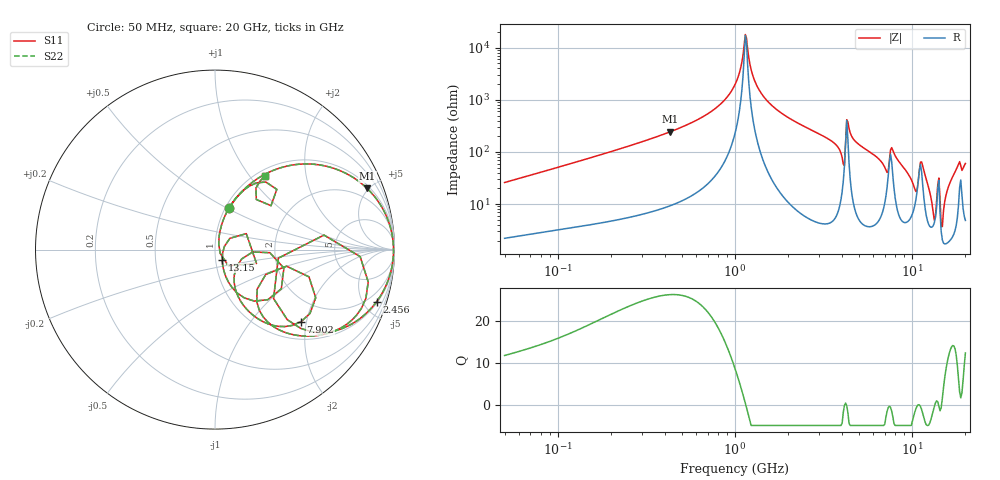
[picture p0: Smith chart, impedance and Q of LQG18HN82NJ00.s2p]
!Murata Part Number: LQG18HN82NJ00
!These Parameters are Measured in Series Mode Connection
!  o--[Z]--o
!Port1  Port2
!  o-------o
!Freq. Start=50[MHz] Stop=20[GHz], 401[Steps]
# Hz S RI R 50
!Freq.(Hz) S11(Real) S11(Imag) S21(Real) S21(Imag) S12(Real) S12(Imag) S22(Real) S22(Imag)
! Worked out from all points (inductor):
!   401 points, 50 MHz to 20 GHz, reference 50 ohm
!   read as one part in series: L = 81.2 nH near 51.52 MHz
!   highest Q = 26.2 at 432.2 MHz (marker M1), where L = 90.1 nH
!   self-resonance near 1.144 GHz
!   S11 on the Smith chart (normalised r, x): 50 MHz: 1.04, +0.52; 2.456 GHz: 1.12, -6.19; 7.902 GHz: 1.41, -1.86; 13.15 GHz: 1.08, -0.12; 20 GHz: 1.10, +1.20
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5e7  0.0802 0.2322  0.9198 -0.2322  0.9198 -0.2322  0.0802 0.2322
1.364002e8  0.3309 0.4439  0.6691 -0.4439  0.6691 -0.4439  0.3309 0.4439
3.721004e8  0.7954 0.3845  0.2046 -0.3845  0.2046 -0.3845  0.7954 0.3845
4.322267e8  0.8479 0.3406  0.1521 -0.3406  0.1521 -0.3406  0.8479 0.3406
1e9  0.9916 0.0499  0.00837 -0.0499  0.00837 -0.0499  0.9916 0.0499
1.161586e9  0.9947 -0.00387  0.00529 0.00387  0.00529 0.00387  0.9947 -0.00387
1.432596e9  0.9886 -0.0804  0.0114 0.0804  0.0114 0.0804  0.9886 -0.0804
2.456456e9  0.9009 -0.2894  0.0991 0.2894  0.0991 0.2894  0.9009 -0.2894
2.728004e9  0.8653 -0.3322  0.1347 0.3322  0.1347 0.3322  0.8653 -0.3322
4.026975e9  0.403 -0.391  0.597 0.391  0.597 0.391  0.403 -0.391
4.275624e9  0.8087 -0.0391  0.1913 0.0391  0.1913 0.0391  0.8087 -0.0391
4.677679e9  0.741 -0.4108  0.259 0.4108  0.259 0.4108  0.741 -0.4108
5.944466e9  0.4661 -0.4792  0.5339 0.4792  0.5339 0.4792  0.4661 -0.4792
7.442007e9  0.3988 -0.0924  0.6012 0.0924  0.6012 0.0924  0.3988 -0.0924
7.901521e9  0.4791 -0.4018  0.5209 0.4018  0.5209 0.4018  0.4791 -0.4018
1.050288e10  0.1188 -0.0988  0.8812 0.0988  0.8812 0.0988  0.1188 -0.0988
1.149051e10  0.2939 -0.2793  0.7061 0.2793  0.7061 0.2793  0.2939 -0.2793
1.314879e10  0.0401 -0.0563  0.9599 0.0563  0.9599 0.0563  0.0401 -0.0563
1.396067e10  0.1744 0.0889  0.8256 -0.0889  0.8256 -0.0889  0.1744 0.0889
1.504638e10  0.0225 0.0695  0.9775 -0.0695  0.9775 -0.0695  0.0225 0.0695
1.670968e10  0.0997 0.2655  0.9003 -0.2655  0.9003 -0.2655  0.0997 0.2655
2e10  0.2808 0.4107  0.7192 -0.4107  0.7192 -0.4107  0.2808 0.4107
